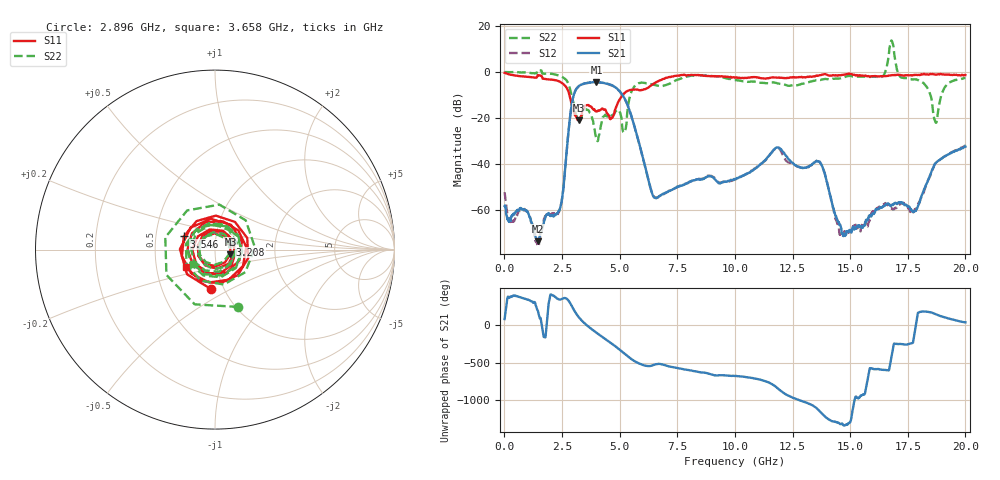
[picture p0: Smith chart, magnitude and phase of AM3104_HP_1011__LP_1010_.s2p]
!Created with skrf (http://scikit-rf.org).
# Hz S RI R 50.0
!freq ReS11 ImS11 ReS21 ImS21 ReS12 ImS12 ReS22 ImS22
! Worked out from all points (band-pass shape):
!   1601 points, 10 MHz to 20 GHz, reference 50 ohm
!   highest |S21| = -4.45 dB at 3.996 GHz (marker M1); lowest = -73.5 dB at 1.459 GHz (marker M2)
!   |S21| within 3 dB of the highest: 3.116 GHz to 4.909 GHz (1.793 GHz wide, 44.7 % of centre)
!   lowest |S11| = -21.0 dB at 3.221 GHz (marker M3), VSWR 1.20, Z = 59.3 - j3.05 ohm
!   |S11| at or under -10 dB: 2.824 GHz to 5.135 GHz (2.311 GHz wide, 58.1 % of centre)
!   |S22| runs from -30.0 to 13.6 dB; largest |S21 - S12| = 0.05
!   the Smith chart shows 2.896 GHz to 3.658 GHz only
!   S11 on the Smith chart (normalised r, x): 2.896 GHz: 0.87, -0.40; 3.208 GHz: 1.18, +0.07; 3.546 GHz: 0.70, +0.11; 3.658 GHz: 0.71, -0.15
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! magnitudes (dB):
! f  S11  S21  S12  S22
! 10 MHz  -0.4  -58.2  -52.2  -0.1
! 1.459 GHz  -1.4  -73.5  -75.2  0.8
! 2.421 GHz  -4.3  -58.9  -58.8  -1.8
! 2.896 GHz  -13.1  -15.9  -15.9  -9.3
! 3.208 GHz  -20.9  -6.3  -6.4  -21.5
! 3.221 GHz  -21.0  -6.2  -6.3  -21.7
! 3.346 GHz  -18.7  -5.5  -5.5  -19.6
! 3.546 GHz  -14.5  -4.9  -4.9  -16.2
! 3.658 GHz  -14.4  -4.7  -4.8  -16.7
! 3.996 GHz  -17.0  -4.5  -4.5  -28.7
! 5.207 GHz  -9.2  -11.4  -11.4  -26.2
! 5.645 GHz  -7.7  -23.7  -23.7  -6.2
! 6.682 GHz  -4.0  -54.2  -54.3  -6.0
! 10.01 GHz  -2.5  -46.6  -46.7  -3.6
! 11.83 GHz  -2.5  -32.8  -32.9  -4.9
! 13.34 GHz  -2.1  -40.2  -40.2  -4.1
! 13.8 GHz  -1.1  -41.3  -41.1  -3.3
! 14.63 GHz  -1.3  -69.1  -71.2  -2.7
! 16.68 GHz  -1.6  -57.4  -58.5  7.2
! 17.83 GHz  -1.3  -60.2  -59.6  -3.2
! 18.7 GHz  -1.2  -39.6  -39.7  -21.7
! 20 GHz  -1.3  -32.4  -32.0  -2.6
